[IBIS Ver] 2.1
[File Name] sprm015.ibs
[File Rev] 0.1
[Date] January 31, 2001
[Source] IBIS Model Generated from PACED 4.40B
[Disclaimer]   Please be aware that in the absence of a written agreement
|   Texas Instruments(TI) assumes no liability for:
|   (1) The accuracy of the IBIS models provided to your company
|   (2) The proper functioning of these Models in your design
|   or for any resulting applications; or
|   (3)Infringement of patents, copyrights or intellectual
|   property rights resulting from your use of these models.
|   TI provides IBIS Models as a service to our customers and
|   therefore reserves the right to limit distribution of the
|   Models.
[Copyright]   Property of Texas Instruments Incorporated.
|   Unauthorized reproduction and/or distribution is strictly.
|   prohibited.
|   This product is protected under copyright law and trade
|   secret law as an unpublished work.
|   Created 1999,(C) Copyright 1999-2000,
|   Texas Instruments Incorporated., All Rights Reserved.
|   These commodities are under the U.S.
|   Government distribution license control. As such,they are
|   not to be re-exported without the prior approval of the U.S.
|   Department of Commerce.
[Component]   c6204_GLW
[Manufacturer]  Texas Instruments
[Package]
|Variable  Typ   Min   Max
R_pkg   0.1438   0.04944   0.2287
L_pkg   5.97E-10 3.88E-10  2.05E-09
C_pkg   7.15E-13 1.71E-13  1.01E-12
[Pin] signal_name   model_name   R_pin   L_pin   C_pin
B10   CLKIN   IDH041   0.1225   1.84E-09   9.36E-13
Y18   CLKOUT1   OUH831   0.1390   1.92E-09   9.36E-13
AB19  CLKOUT2   OUH831   0.1874   2.77E-09   1.41E-12
B12   CLKMODE0   IDH041   0.1332   1.95E-09   9.80E-13
Y5   TMS   IDH041_PS1001   0.1602   2.26E-09   1.08E-12
AA4   TDO   OUH831   0.1581   2.34E-09   1.21E-12
Y4   TDI   IDH041_PS1001   0.1742   2.44E-09   1.14E-12
AB2   TCK   IDH041   0.2108   3.14E-09   1.55E-12
AA3   TRSTz   IDH041_PE1001   0.1728   2.52E-09   1.27E-12
AA5   EMU1   IDH041_OUH831_PE1001  0.1772   2.53E-09   1.19E-12
AB4   EMU0   IDH041_OUH831_PE1001  0.1694   2.55E-09   1.36E-12
J3   RESETz   IDH041   0.1321   1.83E-09   8.34E-13
K2   NMI   IDH041   0.1505   2.14E-09   1.04E-12
U2   EXT_INT7   IDH041_OUI431   0.1584   2.26E-09   1.07E-12
U3   EXT_INT6   IDH041   0.1249   1.79E-09   8.57E-13
W1   EXT_INT5   IDH041_OUI431   0.1600   2.48E-09   1.33E-12
V2   EXT_INT4   IDH041_OUI431   0.1502   2.15E-09   1.03E-12
V1   IACK   IDH041_OUI431   0.1691   2.57E-09   1.37E-12
R3   INUM3   IDH041_OUI431   0.1202   1.75E-09   8.70E-13
T1   INUM2   IDH041_OUI431   0.1672   2.40E-09   1.19E-12
T2   INUM1   IDH041_OUI431   0.1452   2.12E-09   1.06E-12
T3   INUM0   IDH041_OUI431   0.1394   1.93E-09   8.81E-13
Y2   PD   OUI431   0.1689   2.49E-09   1.21E-12
C8   XCLKIN   UBS032   0.1292   1.80E-09   8.21E-13
A8   XFCLK   UBS032   0.1654   2.37E-09   1.13E-12
C13   XD31   UBS032   0.1236   1.78E-09   8.58E-13
A13   XD30   UBS032   0.1497   2.32E-09   1.26E-12
C14   XD29   UBS032   0.1303   1.80E-09   8.24E-13
B14   XD28   UBS032   0.1427   2.08E-09   1.04E-12
B15   XD27   UBS032   0.1384   1.93E-09   8.56E-13
C15   XD26   UBS032   0.0549   6.79E-10   2.17E-13
A15   XD25   UBS032   0.1522   2.31E-09   1.19E-12
B16   XD24   UBS032   0.1618   2.28E-09   1.06E-12
C16   XD23   UBS032   0.1298   1.83E-09   8.66E-13
A17   XD22   UBS032   0.1646   2.41E-09   1.19E-12
B17   XD21   UBS032   0.1511   2.18E-09   1.08E-12
C17   XD20   UBS032   0.1486   2.04E-09   9.48E-13
B18   XD19   UBS032   0.1692   2.49E-09   1.26E-12
A19   XD18   UBS032   0.1830   2.70E-09   1.39E-12
C18   XD17   UBS032   0.1454   2.04E-09   1.01E-12
B19   XD16   UBS032   0.1828   2.65E-09   1.31E-12
C19   XD15   UBS032   0.1574   2.22E-09   1.07E-12
B20   XD14   UBS032   0.1970   2.74E-09   1.29E-12
A21   XD13   UBS032   0.2008   2.94E-09   1.44E-12
C21   XD12   UBS032   0.1833   2.62E-09   1.19E-12
D20   XD11   UBS032   0.1404   1.94E-09   8.79E-13
B22   XD10   UBS032   0.1915   2.73E-09   1.28E-12
D21   XD9   UBS032   0.1646   2.43E-09   1.23E-12
E20   XD8   UBS032   0.1537   2.13E-09   9.65E-13
E21   XD7   UBS032   0.1443   2.05E-09   9.67E-13
D22   XD6   UBS032   0.1776   2.66E-09   1.36E-12
F20   XD5   UBS032   0.1209   1.72E-09   8.14E-13
F21   XD4   UBS032   0.1536   2.13E-09   1.01E-12
E22   XD3   UBS032   0.1900   2.75E-09   1.40E-12
G20   XD2   UBS032   0.1275   1.75E-09   7.96E-13
G21   XD1   UBS032   0.1557   2.24E-09   1.08E-12
G22   XD0   UBS032   0.1627   2.42E-09   1.24E-12
D2   XCE3z   UBS032   0.1905   2.79E-09   1.37E-12
B1   XCE2z   UBS032   0.2287   3.39E-09   1.72E-12
D3   XCE1z   UBS032   0.1987   2.77E-09   1.28E-12
C2   XCE0z   UBS032   0.2072   3.04E-09   1.47E-12
C5   XBE3z/XA5   UBS032   0.1371   1.90E-09   9.02E-13
A4   XBE2z/XA4   UBS032   0.1758   2.57E-09   1.32E-12
B5   XBE1z/XA3   UBS032   0.05437   6.55E-10   1.90E-13
C6   XBE0z/XA2   UBS032   0.1486   2.02E-09   8.94E-13
A6   XOEz   UBS032   0.1679   2.41E-09   1.16E-12
C7   XREz   UBS032   0.1416   1.93E-09   8.51E-13
B7   XWEz/XWAIT   UBS032   0.1514   2.11E-09   1.00E-12
C9   XCSz   UBS032   0.1171   1.69E-09   8.09E-13
B6   XASz   UBS032   0.1723   2.32E-09   1.03E-12
B9   XCNTL   UBS032   0.1437   2.04E-09   9.66E-13
B8   XW/R   UBS032   0.1539   2.09E-09   9.60E-13
C4   XRDY   UBS032   0.1719   2.44E-09   1.16E-12
B4   XBLAST   UBS032   0.1607   2.31E-09   1.11E-12
A10   XBOFF   UBS032   0.1339   2.09E-09   1.12E-12
A2   XHOLD   UBS032   0.2019   2.95E-09   1.43E-12
B3   XHOLDA   UBS032   0.1956   2.71E-09   1.26E-12
Y21   CE3z   OUH831   0.1635   2.37E-09   1.13E-12
W20   CE2z   OUH831   0.1668   2.32E-09   1.04E-12
AA22  CE1z   OUH831   0.1918   2.85E-09   1.45E-12
W21   CE0z   OUH831   0.1823   2.61E-09   1.25E-12
V20   BE3z   OUH831   0.1384   1.94E-09   9.15E-13
V21   BE2z   OUH831   0.1647   2.33E-09   1.10E-12
W22   BE1z   OUH831   0.1617   2.42E-09   1.25E-12
U20   BE0z   OUH831   0.1383   1.93E-09   8.74E-13
H20   EA21   IDH041_OUH831_PE1001  0.1382   1.92E-09   8.49E-13
H21   EA20   IDH041_OUH831_PE1001  0.06215   7.47E-10   2.23E-13
H22   EA19   IDH041_OUH831_PE1001  0.1415   2.11E-09   1.07E-12
J20   EA18   IDH041_OUH831_PE1001  0.1350   1.86E-09   8.35E-13
J21   EA17   IDH041_OUH831   0.1242   1.75E-09   8.21E-13
K21   EA16   IDH041_OUH831   0.1601   2.28E-09   1.10E-12
K20   EA15   IDH041_OUH831   0.1341   1.88E-09   8.62E-13
K22   EA14   IDH041_OUH831   0.1383   2.04E-09   1.03E-12
L21   EA13   IDH041_OUH831   0.1514   2.11E-09   9.86E-13
L20   EA12   IDH041_OUH831   0.1136   1.54E-09   6.95E-13
L22   EA11   IDH041_OUH831   0.1541   2.19E-09   1.06E-12
M20   EA10   IDH041_OUH831   0.1155   1.55E-09   6.81E-13
M21   EA9   IDH041_OUH831   0.1558   2.16E-09   9.72E-13
N22   EA8   IDH041_OUH831   0.1440   2.08E-09   1.02E-12
N20   EA7   IDH041_OUH831   0.1475   1.98E-09   8.55E-13
N21   EA6   IDH041_OUH831   0.1475   2.07E-09   9.56E-13
P21   EA5   IDH041_OUH831   0.1491   2.09E-09   9.63E-13
P20   EA4   IDH041_OUH831   0.1346   1.85E-09   8.01E-13
R22   EA3   IDH041_OUH831   0.0628   7.54E-10   2.27E-13
R21   EA2   IDH041_OUH831   0.1248   1.84E-09   8.98E-13
Y6   ED31   IDH041_OUH831_PE1001  0.1394   1.93E-09   8.72E-13
AA6   ED30   IDH041_OUH831_PE1001  0.1705   2.39E-09   1.10E-12
AB6   ED29   IDH041_OUH831_PE1001  0.1527   2.28E-09   1.19E-12
Y7   ED28   IDH041_OUH831_PE1001  0.1403   1.99E-09   9.40E-13
AA7   ED27   IDH041_OUH831_PE1001  0.1436   2.06E-09   9.97E-13
AB8   ED26   IDH041_OUH831_PE1001  0.1722   2.49E-09   1.22E-12
Y8   ED25   IDH041_OUH831_PE1001  0.1498   2.02E-09   8.77E-13
AA8   ED24   IDH041_OUH831_PE1001  0.1432   2.04E-09   9.97E-13
AA9   ED23   IDH041_OUH831_PE1001  0.1576   2.25E-09   1.07E-12
Y9   ED22   IDH041_OUH831_PE1001  0.1355   1.88E-09   8.57E-13
AB10  ED21   IDH041_OUH831_PE1001  0.1748   2.52E-09   1.27E-12
Y10   ED20   IDH041_OUH831_PE1001  0.1284   1.75E-09   7.52E-13
AA10  ED19   IDH041_OUH831_PE1001  0.1265   1.85E-09   9.03E-13
AA11  ED18   IDH041_OUH831_PE1001  0.1434   2.07E-09   1.01E-12
Y11   ED17   IDH041_OUH831_PE1001  0.1021   1.47E-09   7.23E-13
AB12  ED16   IDH041_OUH831_PE1001  0.1626   2.56E-09   1.45E-12
Y12   ED15   IDH041_OUH831_PE1001  0.09674   1.38E-09   6.65E-13
AA12  ED14   IDH041_OUH831_PE1001  0.1427   2.02E-09   9.45E-13
AA13  ED13   IDH041_OUH831_PE1001  0.1280   1.80E-09   8.26E-13
Y13   ED12   IDH041_OUH831_PE1001  0.1319   1.82E-09   8.16E-13
AB13  ED11   IDH041_OUH831_PE1001  0.1303   1.96E-09   1.04E-12
Y14   ED10   IDH041_OUH831_PE1001  0.1268   1.80E-09   8.42E-13
AA14  ED9   IDH041_OUH831_PE1001  0.1343   1.90E-09   9.21E-13
AA15  ED8   IDH041_OUH831_PE1001  0.1558   2.15E-09   1.02E-12
Y15   ED7   IDH041_OUH831_PE1001  0.1190   1.65E-09   7.66E-13
AB15  ED6   IDH041_OUH831_PE1001  0.1467   2.15E-09   1.08E-12
AA16  ED5   IDH041_OUH831_PE1001  0.1583   2.19E-09   1.05E-12
Y16   ED4   IDH041_OUH831_PE1001  0.1231   1.71E-09   8.12E-13
AB17  ED3   IDH041_OUH831_PE1001  0.1681   2.43E-09   1.22E-12
AA17  ED2   IDH041_OUH831_PE1001  0.1455   2.05E-09   9.72E-13
Y17   ED1   IDH041_OUH831_PE1001  0.0658   7.89E-10   2.39E-13
AA18  ED0   IDH041_OUH831_PE1001  0.1514   2.20E-09   1.05E-12
T21   AREz   OUH831   0.1402   2.04E-09   9.97E-13
R20   AOEz   OUH831   0.1212   1.68E-09   7.75E-13
T22   AWEz   OUH831   0.1689   2.46E-09   1.21E-12
T20   ARDY   IDH041_PE1001   0.1460   1.98E-09   8.71E-13
AA19  SDA10   OUH831   0.1744   2.52E-09   1.26E-12
AB21  SDCASz/SSADSz  OUH831   0.1914   2.78E-09   1.35E-12
Y19   SDRASz/SSOEz   OUH831   0.1501   2.09E-09   9.85E-13
AA20  SDWEz/SSWEz   OUH831   0.1998   2.79E-09   1.33E-12
V22   HOLDz   IDH041   0.1668   2.42E-09   1.24E-12
U21   HOLDAz   OUH831   0.1671   2.29E-09   1.04E-12
F2   TOUT1   OUI431   0.1676   2.35E-09   1.09E-12
F3   TINP1   IDH041_PE1001   0.1617   2.22E-09   9.92E-13
D1   TOUT0   OUI431   0.2055   2.90E-09   1.40E-12
E2   TINP0   IDH041   0.1723   2.40E-09   1.11E-12
V3   DMAC3   IDH041_OUI431_PE1001  0.1445   2.05E-09   9.82E-13
W2   DMAC2   OUI431   0.1734   2.49E-09   1.21E-12
AA1   DMAC1   IDH041_OUI431_PE1001  0.1963   2.95E-09   1.53E-12
W3   DMAC0   OUI431   0.1595   2.22E-09   1.01E-12
K3   CLKS0   IDH041_PE1001   0.1340   1.87E-09   8.45E-13
L2   CLKR0   IDH041_OUI431_PE1001  0.1277   1.94E-09   1.02E-12
K1   CLKX0   IDH041_OUI431_PE1001  0.1474   2.27E-09   1.19E-12
M2   DR0   IDH041_PE1001   0.1115   1.68E-09   8.83E-13
M3   DX0   OUI431   0.1076   1.54E-09   7.22E-13
M1   FSR0   IDH041_OUI431_PE1001  0.133   2.14E-09   1.21E-12
L3   FSX0   IDH041_OUI431_PE1001  0.11   1.62E-09   8.12E-13
E1   CLKS1   IDH041_PE1001   0.1896   2.70E-09   1.31E-12
G2   CLKR1   IDH041_OUI431_PE1001  0.1556   2.18E-09   1.02E-12
G3   CLKX1   IDH041_OUI431_PE1001  0.1463   2.01E-09   8.95E-13
H1   DR1   IDH041_PE1001   0.1741   2.49E-09   1.23E-12
H2   DX1   OUI431   0.1549   2.20E-09   1.05E-12
H3   FSR1   IDH041_OUI431_PE1001  0.1375   1.88E-09   8.27E-13
G1   FSX1   IDH041_OUI431_PE1001  0.1595   2.29E-09   1.15E-12
| End of package information
[Component]   IDH041
[Manufacturer]   Texas Instruments
[Package]
|   typ   min   max
R_pkg   0   0   0
L_pkg   0   0   0
C_pkg   0   0   0
[Pin]   signal_name   model_name   R_pin   L_pin   C_pin
   1   A   IDH041   0   0   0
[Component]   OUH831
[Manufacturer]   Texas Instruments
[Package]
|   typ   min   max
R_pkg   0   0   0
L_pkg   0   0   0
C_pkg   0   0   0
[Pin]   signal_name   model_name   R_pin   L_pin   C_pin
   1   Y   OUH831   0   0   0
[Component]   UIS327
[Manufacturer]   Texas Instruments
[Package]
|   typ   min   max
R_pkg   0   0   0
L_pkg   0   0   0
C_pkg   0   0   0
[Pin]   signal_name   model_name   R_pin   L_pin   C_pin
   1   A   UIS327   0   0   0
[Component]   OUI431
[Manufacturer]   Texas Instruments
[Package]
|   typ   min   max
R_pkg   0   0   0
L_pkg   0   0   0
C_pkg   0   0   0
[Pin]   signal_name   model_name   R_pin   L_pin   C_pin
   1   Y   OUI431   0   0   0
[Component]   UBS032
[Manufacturer]   Texas Instruments
[Package]
|   typ   min   max
R_pkg   0   0   0
L_pkg   0   0   0
C_pkg   0   0   0
[Pin]   signal_name   model_name   R_pin   L_pin   C_pin
   1   Y2   UBS032   0   0   0
[Component]   IDH041_PE1001
[Manufacturer]   Texas Instruments
[Package]
|   typ   min   max
R_pkg   0   0   0
L_pkg   0   0   0
C_pkg   0   0   0
[Pin]   signal_name   model_name   R_pin   L_pin   C_pin
   1   A   IDH041_PE1001   0   0   0
[Component]   IDH041_OUH831_PE1001
[Manufacturer]   Texas Instruments
[Package]
|   typ   min   max
R_pkg   0   0   0
L_pkg   0   0   0
C_pkg   0   0   0
[Pin]   signal_name   model_name   R_pin   L_pin   C_pin
   1   Y   IDH041_OUH831_PE1001   0   0   0
[Component]   IDH041_OUI431
[Manufacturer]   Texas Instruments
[Package]
|   typ   min   max
R_pkg   0   0   0
L_pkg   0   0   0
C_pkg   0   0   0
[Pin]   signal_name   model_name   R_pin   L_pin   C_pin
   1   Y   IDH041_OUI431   0   0   0
[Component]   UIS328
[Manufacturer]   Texas Instruments
[Package]
|   typ   min   max
R_pkg   0   0   0
L_pkg   0   0   0
C_pkg   0   0   0
[Pin]   signal_name   model_name   R_pin   L_pin   C_pin
   1   ZRINGDET   UIS328   0   0   0
[Component]   UIS341
[Manufacturer]   Texas Instruments
[Package]
|   typ   min   max
R_pkg   0   0   0
L_pkg   0   0   0
C_pkg   0   0   0
[Pin]   signal_name   model_name   R_pin   L_pin   C_pin
   1   A   UIS341   0   0   0
[Component]   IDH041_OUH831
[Manufacturer]   Texas Instruments
[Package]
|   typ   min   max
R_pkg   0   0   0
L_pkg   0   0   0
C_pkg   0   0   0
[Pin]   signal_name   model_name   R_pin   L_pin   C_pin
   1   Y   IDH041_OUH831   0   0   0
[Component]   IDH041_PS1001
[Manufacturer]   Texas Instruments
[Package]
|   typ   min   max
R_pkg   0   0   0
L_pkg   0   0   0
C_pkg   0   0   0
[Pin]   signal_name   model_name   R_pin   L_pin   C_pin
   1   A   IDH041_PS1001   0   0   0
[Component]   IDH041_OUI431_PE1001
[Manufacturer]   Texas Instruments
[Package]
|   typ   min   max
R_pkg   0   0   0
L_pkg   0   0   0
C_pkg   0   0   0
[Pin]   signal_name   model_name   R_pin   L_pin   C_pin
   1   Y   IDH041_OUI431_PE1001   0   0   0
| Models and submodels in the file (13): IDH041 (Input), OUH831 (3-state), UIS327 (Input), OUI431 (3-state), UBS032 (I/O), IDH041_PE1001 (Input), IDH041_OUH831_PE1001 (I/O), IDH041_OUI431 (I/O), UIS328 (Input), UIS341 (Input), IDH041_OUH831 (I/O), IDH041_PS1001 (Input), IDH041_OUI431_PE1001 (I/O)
